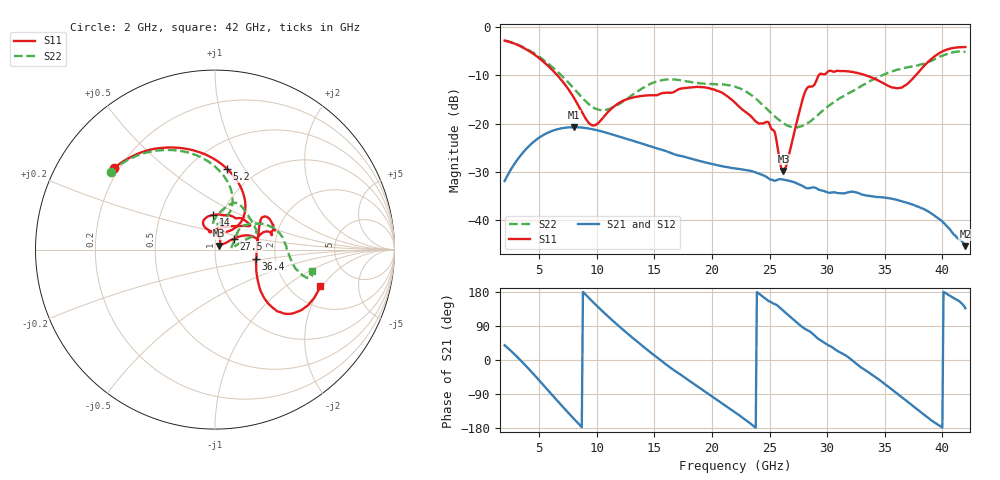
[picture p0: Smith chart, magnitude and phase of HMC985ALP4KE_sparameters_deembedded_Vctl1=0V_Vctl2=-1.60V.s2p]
!s2p File: Measurements: S11, S21, S12, S22
# GHz S dB R 50.0
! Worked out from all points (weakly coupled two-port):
!   401 points, 2 GHz to 42 GHz, reference 50 ohm
!   highest |S21| = -20.72 dB at 8 GHz (marker M1); lowest = -45.3 dB at 42 GHz (marker M2)
!   lowest |S11| = -29.8 dB at 26.2 GHz (marker M3), VSWR 1.07, Z = 52.4 + j2.32 ohm
!   |S11| at or under -10 dB: 6.577 GHz to 29.27 GHz (22.69 GHz wide, 127 % of centre); 33.36 GHz to 37.69 GHz (4.338 GHz wide, 12.2 % of centre)
!   |S22| runs from -20.8 to -2.8 dB; largest |S21 - S12| = 0.00014
!   S11 on the Smith chart (normalised r, x): 2 GHz: 0.18, +0.34; 5.2 GHz: 0.74, +0.84; 14 GHz: 0.91, +0.37; 27.5 GHz: 1.22, +0.15; 36.4 GHz: 1.58, -0.18; 42 GHz: 2.90, -1.91
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2  -2.82 141.1  -31.87 39.1  -31.88 39.1  -2.79 143.3
3.5  -4.14 113.5  -26.24 -4.4  -26.25 -4.4  -4.06 117.9
5.2  -6.84 81.4  -22.57 -60.5  -22.58 -60.5  -6.50 91.5
8  -14.57 46.4  -20.72 -154.8  -20.73 -154.9  -12.69 68.3
8.7  -17.56 52.0  -20.80 -177.2  -20.81 -177.2  -14.54 71.0
9.8  -20.36 87.9  -21.23 149.0  -21.23 149.0  -16.79 82.6
11.9  -15.77 114.1  -22.63 89.9  -22.63 89.9  -16.01 92.8
14  -14.24 92.5  -24.17 36.3  -24.18 36.3  -12.61 77.6
15.4  -13.94 73.0  -25.23 3.0  -25.23 2.9  -11.14 68.8
19.3  -12.46 34.5  -27.93 -81.2  -27.93 -81.2  -11.70 39.0
22  -15.65 52.3  -29.25 -137.7  -29.26 -137.7  -12.35 21.1
25  -20.14 98.2  -31.47 154.4  -31.48 154.3  -17.51 13.6
26.2  -29.77 43.0  -31.57 129.5  -31.57 129.5  -19.91 6.5
27.5  -18.38 29.9  -32.47 95.3  -32.48 95.3  -20.68 7.1
28.1  -13.34 20.8  -33.21 81.6  -33.20 81.7  -20.18 13.0
28.7  -12.30 12.9  -33.21 70.3  -33.21 70.2  -19.20 20.2
31  -9.07 23.3  -34.38 22.4  -34.36 22.3  -14.87 40.3
33.3  -9.95 34.3  -34.81 -26.6  -34.81 -26.5  -11.79 33.9
35.4  -12.27 12.2  -35.44 -72.7  -35.45 -72.7  -9.40 21.9
36.4  -12.58 -12.9  -35.97 -96.3  -35.99 -96.4  -8.63 14.9
39.5  -5.81 -43.3  -39.35 -168.1  -39.33 -168.3  -6.46 -14.2
42  -4.14 -19.0  -45.32 136.5  -45.26 137.7  -5.11 -12.2
